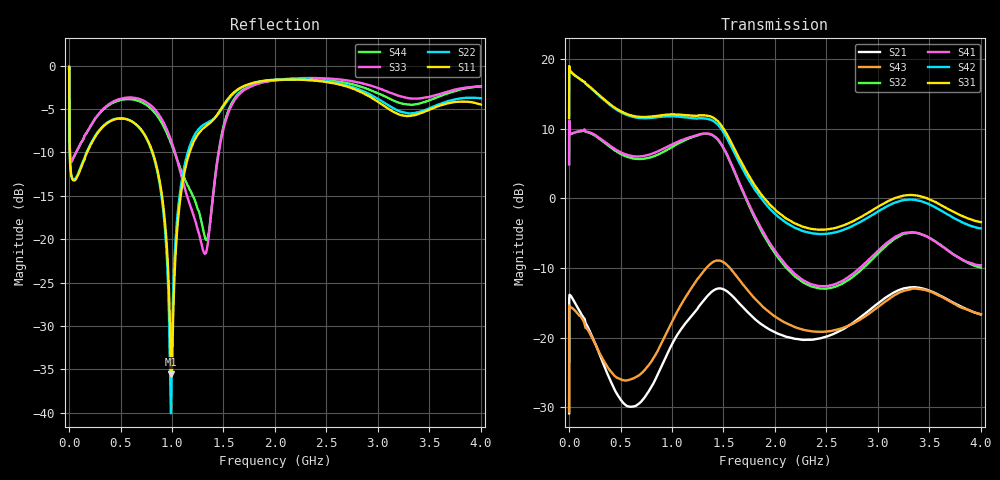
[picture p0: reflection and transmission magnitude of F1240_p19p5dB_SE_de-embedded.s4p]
! Integrated Device Technology
! Corporate Headquarters
! 6024 Silver Creek Valley Road
! San Jose, CA 95138  USA
! Phone:  1-408-284-8200
! Toll Free:  1-800-223-1366
! Webpage:  http://www.idt.com/
! Timing and RF Division
! 515 Groton Road, Suite 102
! Westford, MA 01886-6024
! Device:  F1240
! Description: Dual Intermediate Frequency Digital Variable Gain Amplifier
! Frequency:  10.0 -  500.00 MHz
! Package:  5x5 mm QFN Plastic Package: 32 pin
! Ports:  8 RF, 20 DC
!  Pin  1  = GA3 / Data  Pin 17  = RF OUT_B+
!  Pin  2  = GA4 / CLK  Pin 18  = RF OUT_B-
!  Pin  3  = GA5  Pin 19  = STBY_B
!  Pin  4  = VMODE  Pin 20  = Ground
!  Pin  5  = No Connect  Pin 21  = Ground
!  Pin  6  = GB5  Pin 22  = STB_A
!  Pin  7  = GB4  Pin 23  = RF OUT_A-  = Port 4
!  Pin  8  = GB3  Pin 24  = RF OUT_A+  = Port 3
!  Pin  9  = GB2  Pin 25  = GA0
!  Pin 10  = GB1  Pin 26  = ISET_A
!  Pin 11  = RF IN_B+  Pin 27  = VCC
!  Pin 12  = RF IN_B-  Pin 28  = Ground
!  Pin 13  = Ground  Pin 29  = RF IN_A-  = Port 2
!  Pin 14  = VCC  Pin 30  = RF IN_A+  = Port 1
!  Pin 15  = ISET_B  Pin 31  = GA1
!  Pin 16  = GB0  Pin 32  = GA2 / CSb
! Gain  = +19.5 dB
! State  = 1
! Voltage  = +5.00 V
! Current  = 85.292 mA (one channel only)
! Temperture  =  +25 C
! Test Date  =  2017-10-18
! Board  =  EB4031
! Data:  The device was measured on a custom evaluation board which has
!  individual transmission lines to the RF pins.  Data was collected
!  using a calibrated network analyzer.  The evaluation board was
!  de-embedded using Automatic Fixture Removal.
!  The reference plane is the edge of the package pin.
!  Only Channel A was measured.
!  This data is in single-ended operation.  If your needs are balanced
!  or differential S-parameters then this file needs to be used a
!  linear simulator.
! File Date:  2017-11-10  MJV
! Note:
!  Integrated Device Technology supplies this data as a sample of measured
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# Hz S dB R 100
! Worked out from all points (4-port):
!   410 points, 500 kHz to 4 GHz, reference 100 ohm
!   strongest paths, dB at 500 kHz, 930 MHz, 1.96 GHz, 2.98 GHz, 4 GHz:
!     S31: 11.6, 12.0, -1.0, -1.4, -3.4
!     S42: 11.5, 11.8, -1.6, -2.1, -4.3
!     S41: 4.9, 7.2, -6.6, -7.8, -9.6
!     S32: 4.9, 6.8, -7.0, -8.2, -9.9
!     S43: -30.6, -19.8, -16.5, -15.8, -16.6
!     S21: -30.9, -23.1, -18.9, -15.3, -16.7
!   lowest |S11| = -35.6 dB at 990 MHz (marker M1), VSWR 1.03, Z = 96.8 + j0.729 ohm
!   |S11| at or under -10 dB: 7.662 MHz to 174.7 MHz (167.1 MHz wide, 183 % of centre); 811.8 MHz to 1.17 GHz (358.4 MHz wide, 36.2 % of centre)
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500000  -0.27 -6.9  -30.59 36.4  -27.66 69.4  -64.66 69.1
        -30.86 36.8  -0.26 -6.9  -64.73 71.7  -27.65 70.5
        11.56 -105.7  4.92 72.5  -0.39 0.5  -30.68 -179.9
        4.93 73.6  11.54 -104.6  -30.63 179.8  -0.40 2.8
3500000  -6.51 -47.2  -13.92 15.2  -22.06 6.0  -38.87 40.0
         -13.92 15.1  -6.49 -47.3  -38.84 40.3  -22.06 6.1
         18.77 -170.7  9.79 0.9  -6.17 -41.6  -15.45 24.6
         9.77 0.9  18.76 -170.5  -15.42 24.5  -6.22 -41.5
2.1e8  -9.13 -108.0  -19.34 -113.8  -24.82 -52.0  -33.31 8.6
       -19.36 -112.5  -9.00 -109.9  -33.35 8.6  -24.83 -51.9
       15.93 106.7  9.35 -62.4  -6.92 -78.2  -19.09 -121.3
       9.43 -62.3  15.86 105.8  -19.63 -120.2  -6.95 -77.5
5.5e8  -6.15 -169.3  -29.07 99.9  -26.44 -105.0  -27.54 -58.9
       -29.69 98.9  -6.13 -170.6  -27.71 -57.8  -26.60 -105.4
       12.19 21.9  6.05 -146.4  -3.69 -148.9  -24.80 98.0
       6.32 -147.3  12.05 20.7  -26.16 77.9  -3.87 -148.2
9.9e8  -35.58 166.9  -19.54 -24.8  -23.12 165.6  -22.43 -161.5
       -21.22 -23.6  -40.08 -129.2  -22.79 -157.6  -23.55 165.2
       12.07 -82.6  7.29 120.0  -8.60 149.3  -16.24 -2.9
       7.69 115.0  11.81 -84.5  -18.02 -24.7  -8.93 155.9
1.5e9  -4.54 -134.3  -13.16 165.6  -31.50 46.3  -23.39 67.4
       -13.05 170.9  -4.69 -136.0  -23.48 73.4  -33.90 37.5
       10.03 115.3  7.20 -61.5  -7.27 -102.7  -8.67 166.6
       7.27 -66.6  9.50 113.8  -9.16 159.4  -6.96 -106.4
4e9  -4.48 -159.5  -16.71 51.5  -22.08 -31.3  -19.18 -48.2
     -16.68 50.9  -3.75 -152.5  -21.83 -29.4  -25.76 -9.9
     -3.40 -7.1  -9.93 -153.4  -2.42 -135.6  -14.37 88.6
     -9.61 -163.3  -4.31 1.5  -16.63 62.4  -2.38 -140.1
